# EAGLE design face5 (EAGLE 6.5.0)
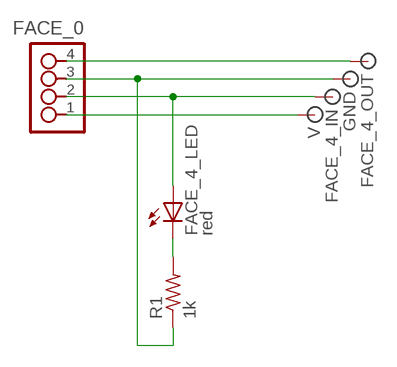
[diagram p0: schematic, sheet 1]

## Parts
FACE_0  4_PIN_HEADER  [SMT_PINS_4]
FACE_4_IN  SIGNAL  [PAD.2]
FACE_4_LED  red  LED1206  [1206]
FACE_4_OUT  SIGNAL  [PAD.2]
GND  SIGNAL  [PAD.2]
R1  1k  RESISTOR1206  [1206]
V  SIGNAL  [PAD.2]

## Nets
N$1: FACE_0.3 GND.P$1 R1.1
N$2: FACE_0.1 V.P$1
N$3: FACE_0.2 FACE_4_IN.P$1 FACE_4_LED.1(A)
N$5: FACE_4_LED.2(C) R1.2
N$6: FACE_0.4 FACE_4_OUT.P$1

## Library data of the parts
FACE_0 = ot:4_PIN_HEADER
FACE_4_IN FACE_4_OUT GND V = ot:SIGNAL: Signal
FACE_4_LED = 01_FAB_Hello:LED
R1 = 01_FAB_Hello:RESISTOR

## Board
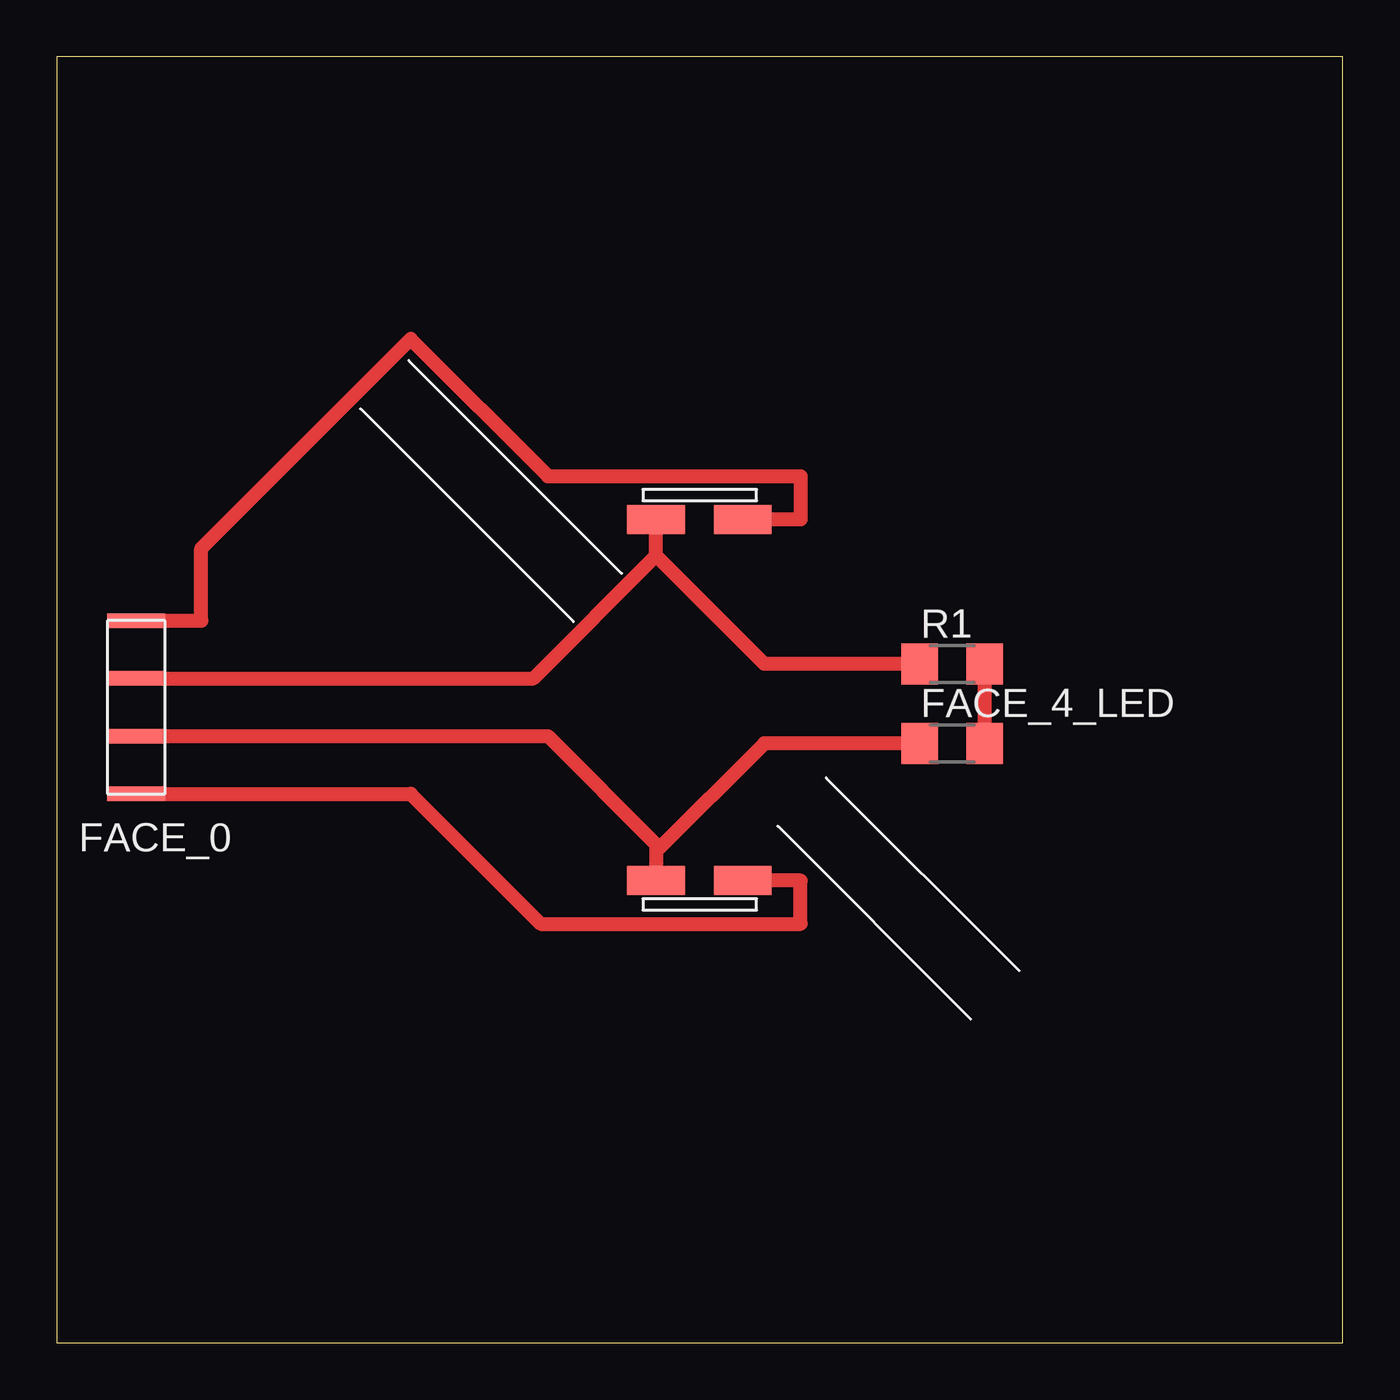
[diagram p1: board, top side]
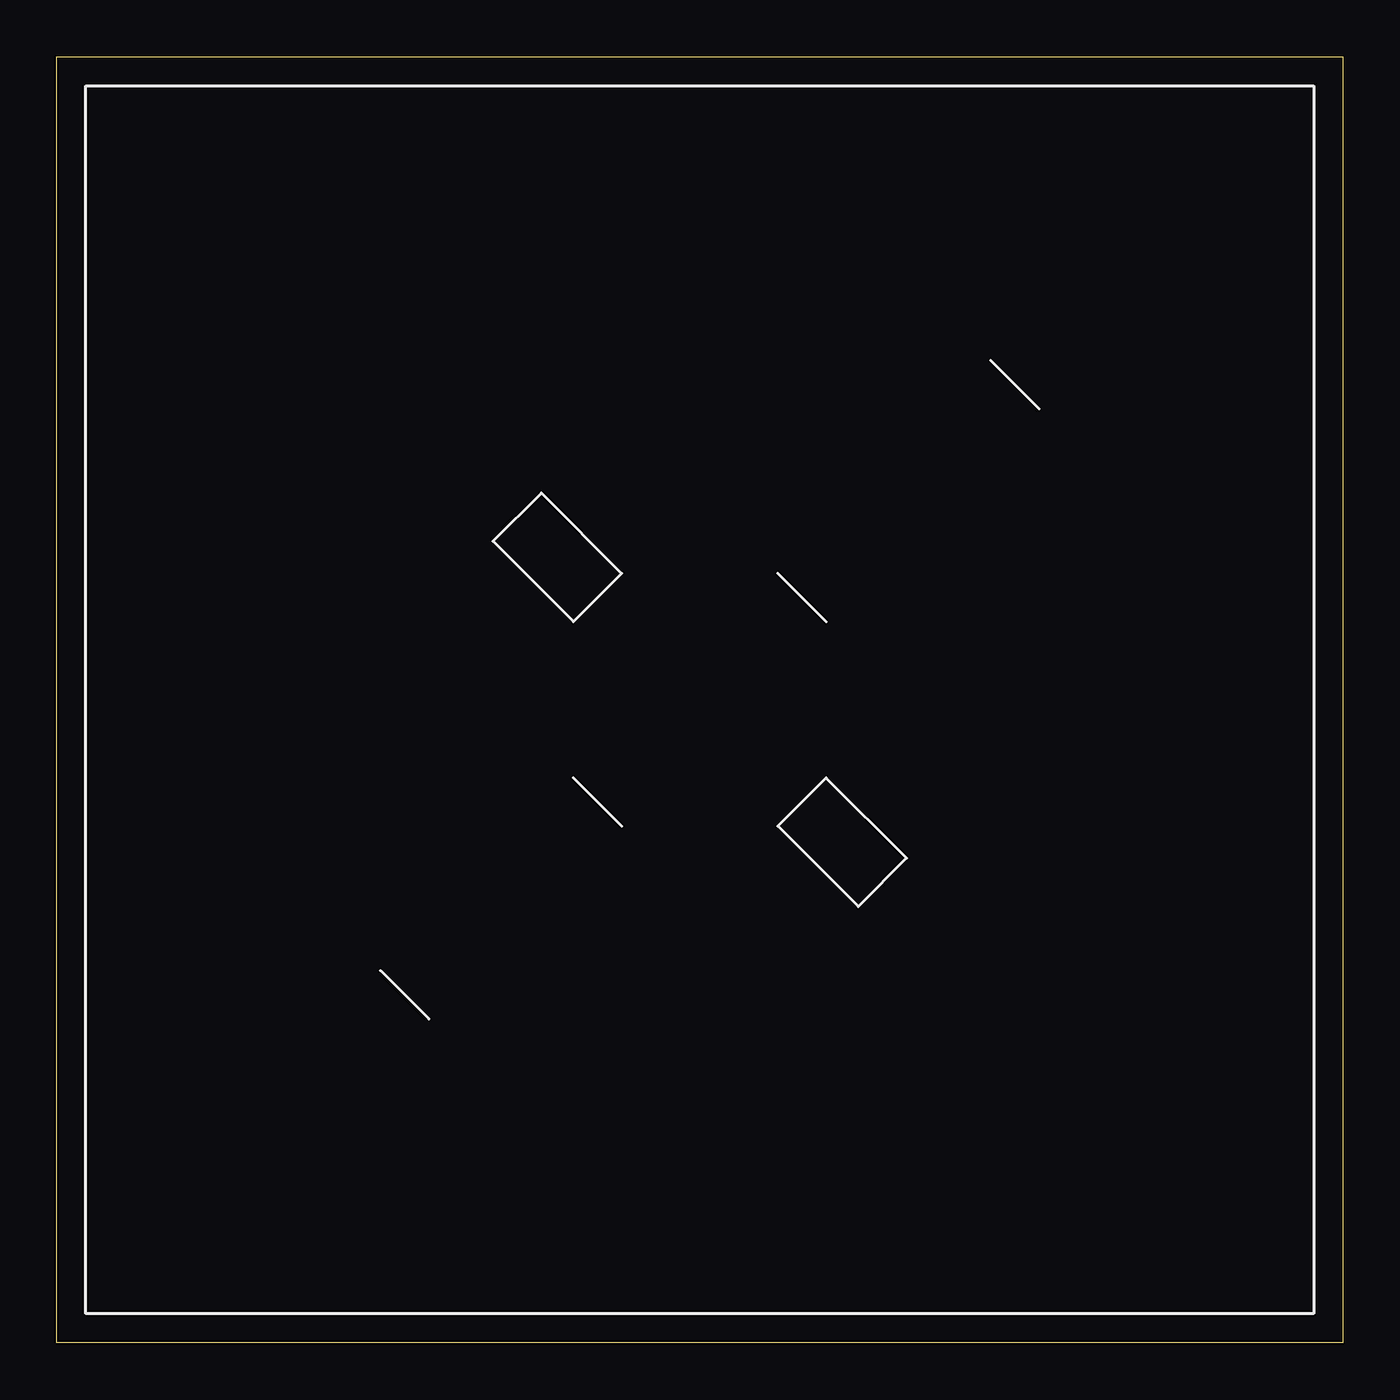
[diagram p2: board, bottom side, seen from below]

Size 56.54 x 56.54 mm. Coordinates in mm from the lower left corner, seen from the top.
Outline: 0,0 56.54,0 56.54,56.54 0,56.54 0,0
Copper layers (1*16): Top 0.035mm / dielectric 1.5mm / Bottom 0.035mm
Design rules "default": minimum track width 10mil, minimum drill 24mil, track to track 8mil, track to pad 8mil, pad to pad 8mil, via to via 8mil, smd to smd 8mil, copper to edge 40mil, drill to drill 8mil, minimum pad ring 10mil, minimum via ring 8mil, stop-mask expansion 4mil, vias tented up to drill 0mil, thermal gap 10mil

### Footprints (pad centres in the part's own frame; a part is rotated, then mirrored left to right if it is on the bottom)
SMT_PINS_4 = smd 2.54 x 0.635: 1 0,0; 2 0,2.54; 3 0,5.08; 4 0,7.62
PAD.2 = smd 2.54 x 1.27: P$1 0,0
1206 = smd 1.6 x 1.803: 1 -1.422,0; 2 1.422,0

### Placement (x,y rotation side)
FACE_0  3.49,24.13 0 top
FACE_4_IN  26.35,20.32 0 top
FACE_4_LED  39.37,26.35 0 top
FACE_4_OUT  30.16,36.2 0 top
GND  26.35,36.2 0 top
R1  39.37,29.84 0 top
U$1  [CUBE_POS]  1.27,1.27 0 top
V  30.16,20.32 0 top

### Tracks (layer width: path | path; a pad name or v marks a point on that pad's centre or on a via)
N$1
  Top 0.61: FACE_0.3 20.95,29.21 26.35,34.61 | 26.35,34.61 GND.P$1 | R1.1 31.11,29.84 26.35,34.61
N$2
  Top 0.61: FACE_0.1 15.56,24.13 21.27,18.41 32.7,18.41 32.7,20.32 V.P$1
N$3
  Top 0.61: FACE_0.2 21.59,26.67 26.35,21.91 26.35,21.59 | 26.35,21.59 FACE_4_IN.P$1 | FACE_4_LED.1 31.11,26.35 26.35,21.59
N$5
  Top 0.61: R1.2 FACE_4_LED.2
N$6
  Top 0.61: FACE_0.4 6.35,31.75 6.35,34.92 15.56,44.13 21.59,38.1 32.7,38.1 32.7,36.2 FACE_4_OUT.P$1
